DATA_BLOCK "IMAC_TANK_RECORD"
TITLE = TANK_RECORD
AUTHOR : HottendU
FAMILY : IMAC
VERSION : 0.2


  STRUCT
   TANK_No001 : STRUCT
    PCONF : STRUCT
     ObjInput : INT  := 1511;	//IMAC L (AvEdit) Objectnumber of pressure/level transmitter, Unit [m] or [bar]
     ObjTemp : INT  := 1512;	//IMAC L (AvEdit) Objectnumber of temperature transmitter
     SklRefNo : BYTE  := B#16#2;	//IMAC L Scaling Group No (AvEdit) user for Tank Table (x=Level, y=Volume)
     Offset : REAL ;	//Offset of pressure transmitter from bottom of tank
     LL_XTsub : REAL ;	//Low limit operator input tank temperature
     HL_XTsub : REAL  := 1.500000e+002;	//High limit operator input tank temperature
     LL_XDensity : REAL ;	//Low limit operator input density (t ref)
     HL_XDensity : REAL  := 5.000000e+000;	//High limit operator input density (t ref)
     LL_XRefTemp : REAL ;	//Low limit operator input reference temperature
     HL_XRefTemp : REAL  := 1.500000e+002;	//High limit operator input reference temperature
     LL_XVEC : REAL ;	//Low limit operator input volume expansion coefficiency
     HL_XVEC : REAL  := 5.000000e+000;	//High limit operator input volume expansion coefficiency
     Modeswitches : STRUCT
      M0_SensorConfiguration : BOOL ;	// 0: Pressure Sensor;  1: Level Sensor
      M1_TemperatureComp : BOOL  := TRUE;	// 0: without Compensation;   1: with compensation
      M2 : BOOL ;	//
      M3 : BOOL ;	//
      M4 : BOOL ;	//
      M5 : BOOL ;	//
      M6 : BOOL ;
      M7 : BOOL ;	//
      M8 : BOOL ;	//
      M9 : BOOL ;	//
      M10 : BOOL ;
      M11 : BOOL ;
      M12 : BOOL ;
      M13 : BOOL ;
      M14 : BOOL ;
      M15 : BOOL ;	//
     END_STRUCT ;
    END_STRUCT ;
   END_STRUCT ;
   TANK_No002 : STRUCT
    PCONF : STRUCT
     ObjInput : INT ;	//IMAC L (AvEdit) Objectnumber of pressure/level transmitter, Unit [m] or [bar]
     ObjTemp : INT ;	//IMAC L (AvEdit) Objectnumber of temperature transmitter
     SklRefNo : BYTE ;	//IMAC L Scaling Group No (AvEdit) user for Tank Table (x=Level, y=Volume)
     Offset : REAL ;	//Offset of pressure transmitter from bottom of tank
     LL_XTsub : REAL ;	//Low limit operator input tank temperature
     HL_XTsub : REAL  := 1.500000e+002;	//High limit operator input tank temperature
     LL_XDensity : REAL ;	//Low limit operator input density (t ref)
     HL_XDensity : REAL  := 5.000000e+000;	//High limit operator input density (t ref)
     LL_XRefTemp : REAL ;	//Low limit operator input reference temperature
     HL_XRefTemp : REAL  := 1.500000e+002;	//High limit operator input reference temperature
     LL_XVEC : REAL ;	//Low limit operator input volume expansion coefficiency
     HL_XVEC : REAL  := 5.000000e+000;	//High limit operator input volume expansion coefficiency
     Modeswitches : STRUCT
      M0_SensorConfiguration : BOOL ;	// 0: Pressure Sensor;  1: Level Sensor
      M1_TemperatureComp : BOOL ;	// 0: without Compensation;   1: with compensation
      M2 : BOOL ;	//
      M3 : BOOL ;	//
      M4 : BOOL ;	//
      M5 : BOOL ;	//
      M6 : BOOL ;
      M7 : BOOL ;	//
      M8 : BOOL ;	//
      M9 : BOOL ;	//
      M10 : BOOL ;
      M11 : BOOL ;
      M12 : BOOL ;
      M13 : BOOL ;
      M14 : BOOL ;
      M15 : BOOL ;	//
     END_STRUCT ;
    END_STRUCT ;
   END_STRUCT ;
   TANK_No003 : STRUCT
    PCONF : STRUCT
     ObjInput : INT ;	//IMAC L (AvEdit) Objectnumber of pressure/level transmitter, Unit [m] or [bar]
     ObjTemp : INT ;	//IMAC L (AvEdit) Objectnumber of temperature transmitter
     SklRefNo : BYTE ;	//IMAC L Scaling Group No (AvEdit) user for Tank Table (x=Level, y=Volume)
     Offset : REAL ;	//Offset of pressure transmitter from bottom of tank
     LL_XTsub : REAL ;	//Low limit operator input tank temperature
     HL_XTsub : REAL  := 1.500000e+002;	//High limit operator input tank temperature
     LL_XDensity : REAL ;	//Low limit operator input density (t ref)
     HL_XDensity : REAL  := 5.000000e+000;	//High limit operator input density (t ref)
     LL_XRefTemp : REAL ;	//Low limit operator input reference temperature
     HL_XRefTemp : REAL  := 1.500000e+002;	//High limit operator input reference temperature
     LL_XVEC : REAL ;	//Low limit operator input volume expansion coefficiency
     HL_XVEC : REAL  := 5.000000e+000;	//High limit operator input volume expansion coefficiency
     Modeswitches : STRUCT
      M0_SensorConfiguration : BOOL ;	// 0: Pressure Sensor;  1: Level Sensor
      M1_TemperatureComp : BOOL ;	// 0: without Compensation;   1: with compensation
      M2 : BOOL ;	//
      M3 : BOOL ;	//
      M4 : BOOL ;	//
      M5 : BOOL ;	//
      M6 : BOOL ;
      M7 : BOOL ;	//
      M8 : BOOL ;	//
      M9 : BOOL ;	//
      M10 : BOOL ;
      M11 : BOOL ;
      M12 : BOOL ;
      M13 : BOOL ;
      M14 : BOOL ;
      M15 : BOOL ;	//
     END_STRUCT ;
    END_STRUCT ;
   END_STRUCT ;
   TANK_No004 : STRUCT
    PCONF : STRUCT
     ObjInput : INT ;	//IMAC L (AvEdit) Objectnumber of pressure/level transmitter, Unit [m] or [bar]
     ObjTemp : INT ;	//IMAC L (AvEdit) Objectnumber of temperature transmitter
     SklRefNo : BYTE ;	//IMAC L Scaling Group No (AvEdit) user for Tank Table (x=Level, y=Volume)
     Offset : REAL ;	//Offset of pressure transmitter from bottom of tank
     LL_XTsub : REAL ;	//Low limit operator input tank temperature
     HL_XTsub : REAL  := 1.500000e+002;	//High limit operator input tank temperature
     LL_XDensity : REAL ;	//Low limit operator input density (t ref)
     HL_XDensity : REAL  := 5.000000e+000;	//High limit operator input density (t ref)
     LL_XRefTemp : REAL ;	//Low limit operator input reference temperature
     HL_XRefTemp : REAL  := 1.500000e+002;	//High limit operator input reference temperature
     LL_XVEC : REAL ;	//Low limit operator input volume expansion coefficiency
     HL_XVEC : REAL  := 5.000000e+000;	//High limit operator input volume expansion coefficiency
     Modeswitches : STRUCT
      M0_SensorConfiguration : BOOL ;	// 0: Pressure Sensor;  1: Level Sensor
      M1_TemperatureComp : BOOL ;	// 0: without Compensation;   1: with compensation
      M2 : BOOL ;	//
      M3 : BOOL ;	//
      M4 : BOOL ;	//
      M5 : BOOL ;	//
      M6 : BOOL ;
      M7 : BOOL ;	//
      M8 : BOOL ;	//
      M9 : BOOL ;	//
      M10 : BOOL ;
      M11 : BOOL ;
      M12 : BOOL ;
      M13 : BOOL ;
      M14 : BOOL ;
      M15 : BOOL ;	//
     END_STRUCT ;
    END_STRUCT ;
   END_STRUCT ;
   TANK_No005 : STRUCT
    PCONF : STRUCT
     ObjInput : INT ;	//IMAC L (AvEdit) Objectnumber of pressure/level transmitter, Unit [m] or [bar]
     ObjTemp : INT ;	//IMAC L (AvEdit) Objectnumber of temperature transmitter
     SklRefNo : BYTE ;	//IMAC L Scaling Group No (AvEdit) user for Tank Table (x=Level, y=Volume)
     Offset : REAL ;	//Offset of pressure transmitter from bottom of tank
     LL_XTsub : REAL ;	//Low limit operator input tank temperature
     HL_XTsub : REAL  := 1.500000e+002;	//High limit operator input tank temperature
     LL_XDensity : REAL ;	//Low limit operator input density (t ref)
     HL_XDensity : REAL  := 5.000000e+000;	//High limit operator input density (t ref)
     LL_XRefTemp : REAL ;	//Low limit operator input reference temperature
     HL_XRefTemp : REAL  := 1.500000e+002;	//High limit operator input reference temperature
     LL_XVEC : REAL ;	//Low limit operator input volume expansion coefficiency
     HL_XVEC : REAL  := 5.000000e+000;	//High limit operator input volume expansion coefficiency
     Modeswitches : STRUCT
      M0_SensorConfiguration : BOOL ;	// 0: Pressure Sensor;  1: Level Sensor
      M1_TemperatureComp : BOOL ;	// 0: without Compensation;   1: with compensation
      M2 : BOOL ;	//
      M3 : BOOL ;	//
      M4 : BOOL ;	//
      M5 : BOOL ;	//
      M6 : BOOL ;
      M7 : BOOL ;	//
      M8 : BOOL ;	//
      M9 : BOOL ;	//
      M10 : BOOL ;
      M11 : BOOL ;
      M12 : BOOL ;
      M13 : BOOL ;
      M14 : BOOL ;
      M15 : BOOL ;	//
     END_STRUCT ;
    END_STRUCT ;
   END_STRUCT ;
   TANK_No006 : STRUCT
    PCONF : STRUCT
     ObjInput : INT ;	//IMAC L (AvEdit) Objectnumber of pressure/level transmitter, Unit [m] or [bar]
     ObjTemp : INT ;	//IMAC L (AvEdit) Objectnumber of temperature transmitter
     SklRefNo : BYTE ;	//IMAC L Scaling Group No (AvEdit) user for Tank Table (x=Level, y=Volume)
     Offset : REAL ;	//Offset of pressure transmitter from bottom of tank
     LL_XTsub : REAL ;	//Low limit operator input tank temperature
     HL_XTsub : REAL  := 1.500000e+002;	//High limit operator input tank temperature
     LL_XDensity : REAL ;	//Low limit operator input density (t ref)
     HL_XDensity : REAL  := 5.000000e+000;	//High limit operator input density (t ref)
     LL_XRefTemp : REAL ;	//Low limit operator input reference temperature
     HL_XRefTemp : REAL  := 1.500000e+002;	//High limit operator input reference temperature
     LL_XVEC : REAL ;	//Low limit operator input volume expansion coefficiency
     HL_XVEC : REAL  := 5.000000e+000;	//High limit operator input volume expansion coefficiency
     Modeswitches : STRUCT
      M0_SensorConfiguration : BOOL ;	// 0: Pressure Sensor;  1: Level Sensor
      M1_TemperatureComp : BOOL ;	// 0: without Compensation;   1: with compensation
      M2 : BOOL ;	//
      M3 : BOOL ;	//
      M4 : BOOL ;	//
      M5 : BOOL ;	//
      M6 : BOOL ;
      M7 : BOOL ;	//
      M8 : BOOL ;	//
      M9 : BOOL ;	//
      M10 : BOOL ;
      M11 : BOOL ;
      M12 : BOOL ;
      M13 : BOOL ;
      M14 : BOOL ;
      M15 : BOOL ;	//
     END_STRUCT ;
    END_STRUCT ;
   END_STRUCT ;
   TANK_No007 : STRUCT
    PCONF : STRUCT
     ObjInput : INT ;	//IMAC L (AvEdit) Objectnumber of pressure/level transmitter, Unit [m] or [bar]
     ObjTemp : INT ;	//IMAC L (AvEdit) Objectnumber of temperature transmitter
     SklRefNo : BYTE ;	//IMAC L Scaling Group No (AvEdit) user for Tank Table (x=Level, y=Volume)
     Offset : REAL ;	//Offset of pressure transmitter from bottom of tank
     LL_XTsub : REAL ;	//Low limit operator input tank temperature
     HL_XTsub : REAL  := 1.500000e+002;	//High limit operator input tank temperature
     LL_XDensity : REAL ;	//Low limit operator input density (t ref)
     HL_XDensity : REAL  := 5.000000e+000;	//High limit operator input density (t ref)
     LL_XRefTemp : REAL ;	//Low limit operator input reference temperature
     HL_XRefTemp : REAL  := 1.500000e+002;	//High limit operator input reference temperature
     LL_XVEC : REAL ;	//Low limit operator input volume expansion coefficiency
     HL_XVEC : REAL  := 5.000000e+000;	//High limit operator input volume expansion coefficiency
     Modeswitches : STRUCT
      M0_SensorConfiguration : BOOL ;	// 0: Pressure Sensor;  1: Level Sensor
      M1_TemperatureComp : BOOL ;	// 0: without Compensation;   1: with compensation
      M2 : BOOL ;	//
      M3 : BOOL ;	//
      M4 : BOOL ;	//
      M5 : BOOL ;	//
      M6 : BOOL ;
      M7 : BOOL ;	//
      M8 : BOOL ;	//
      M9 : BOOL ;	//
      M10 : BOOL ;
      M11 : BOOL ;
      M12 : BOOL ;
      M13 : BOOL ;
      M14 : BOOL ;
      M15 : BOOL ;	//
     END_STRUCT ;
    END_STRUCT ;
   END_STRUCT ;
   TANK_No008 : STRUCT
    PCONF : STRUCT
     ObjInput : INT ;	//IMAC L (AvEdit) Objectnumber of pressure/level transmitter, Unit [m] or [bar]
     ObjTemp : INT ;	//IMAC L (AvEdit) Objectnumber of temperature transmitter
     SklRefNo : BYTE ;	//IMAC L Scaling Group No (AvEdit) user for Tank Table (x=Level, y=Volume)
     Offset : REAL ;	//Offset of pressure transmitter from bottom of tank
     LL_XTsub : REAL ;	//Low limit operator input tank temperature
     HL_XTsub : REAL  := 1.500000e+002;	//High limit operator input tank temperature
     LL_XDensity : REAL ;	//Low limit operator input density (t ref)
     HL_XDensity : REAL  := 5.000000e+000;	//High limit operator input density (t ref)
     LL_XRefTemp : REAL ;	//Low limit operator input reference temperature
     HL_XRefTemp : REAL  := 1.500000e+002;	//High limit operator input reference temperature
     LL_XVEC : REAL ;	//Low limit operator input volume expansion coefficiency
     HL_XVEC : REAL  := 5.000000e+000;	//High limit operator input volume expansion coefficiency
     Modeswitches : STRUCT
      M0_SensorConfiguration : BOOL ;	// 0: Pressure Sensor;  1: Level Sensor
      M1_TemperatureComp : BOOL ;	// 0: without Compensation;   1: with compensation
      M2 : BOOL ;	//
      M3 : BOOL ;	//
      M4 : BOOL ;	//
      M5 : BOOL ;	//
      M6 : BOOL ;
      M7 : BOOL ;	//
      M8 : BOOL ;	//
      M9 : BOOL ;	//
      M10 : BOOL ;
      M11 : BOOL ;
      M12 : BOOL ;
      M13 : BOOL ;
      M14 : BOOL ;
      M15 : BOOL ;	//
     END_STRUCT ;
    END_STRUCT ;
   END_STRUCT ;
   TANK_No009 : STRUCT
    PCONF : STRUCT
     ObjInput : INT ;	//IMAC L (AvEdit) Objectnumber of pressure/level transmitter, Unit [m] or [bar]
     ObjTemp : INT ;	//IMAC L (AvEdit) Objectnumber of temperature transmitter
     SklRefNo : BYTE ;	//IMAC L Scaling Group No (AvEdit) user for Tank Table (x=Level, y=Volume)
     Offset : REAL ;	//Offset of pressure transmitter from bottom of tank
     LL_XTsub : REAL ;	//Low limit operator input tank temperature
     HL_XTsub : REAL  := 1.500000e+002;	//High limit operator input tank temperature
     LL_XDensity : REAL ;	//Low limit operator input density (t ref)
     HL_XDensity : REAL  := 5.000000e+000;	//High limit operator input density (t ref)
     LL_XRefTemp : REAL ;	//Low limit operator input reference temperature
     HL_XRefTemp : REAL  := 1.500000e+002;	//High limit operator input reference temperature
     LL_XVEC : REAL ;	//Low limit operator input volume expansion coefficiency
     HL_XVEC : REAL  := 5.000000e+000;	//High limit operator input volume expansion coefficiency
     Modeswitches : STRUCT
      M0_SensorConfiguration : BOOL ;	// 0: Pressure Sensor;  1: Level Sensor
      M1_TemperatureComp : BOOL ;	// 0: without Compensation;   1: with compensation
      M2 : BOOL ;	//
      M3 : BOOL ;	//
      M4 : BOOL ;	//
      M5 : BOOL ;	//
      M6 : BOOL ;
      M7 : BOOL ;	//
      M8 : BOOL ;	//
      M9 : BOOL ;	//
      M10 : BOOL ;
      M11 : BOOL ;
      M12 : BOOL ;
      M13 : BOOL ;
      M14 : BOOL ;
      M15 : BOOL ;	//
     END_STRUCT ;
    END_STRUCT ;
   END_STRUCT ;
   TANK_No0010 : STRUCT
    PCONF : STRUCT
     ObjInput : INT ;	//IMAC L (AvEdit) Objectnumber of pressure/level transmitter, Unit [m] or [bar]
     ObjTemp : INT ;	//IMAC L (AvEdit) Objectnumber of temperature transmitter
     SklRefNo : BYTE ;	//IMAC L Scaling Group No (AvEdit) user for Tank Table (x=Level, y=Volume)
     Offset : REAL ;	//Offset of pressure transmitter from bottom of tank
     LL_XTsub : REAL ;	//Low limit operator input tank temperature
     HL_XTsub : REAL  := 1.500000e+002;	//High limit operator input tank temperature
     LL_XDensity : REAL ;	//Low limit operator input density (t ref)
     HL_XDensity : REAL  := 5.000000e+000;	//High limit operator input density (t ref)
     LL_XRefTemp : REAL ;	//Low limit operator input reference temperature
     HL_XRefTemp : REAL  := 1.500000e+002;	//High limit operator input reference temperature
     LL_XVEC : REAL ;	//Low limit operator input volume expansion coefficiency
     HL_XVEC : REAL  := 5.000000e+000;	//High limit operator input volume expansion coefficiency
     Modeswitches : STRUCT
      M0_SensorConfiguration : BOOL ;	// 0: Pressure Sensor;  1: Level Sensor
      M1_TemperatureComp : BOOL ;	// 0: without Compensation;   1: with compensation
      M2 : BOOL ;	//
      M3 : BOOL ;	//
      M4 : BOOL ;	//
      M5 : BOOL ;	//
      M6 : BOOL ;
      M7 : BOOL ;	//
      M8 : BOOL ;	//
      M9 : BOOL ;	//
      M10 : BOOL ;
      M11 : BOOL ;
      M12 : BOOL ;
      M13 : BOOL ;
      M14 : BOOL ;
      M15 : BOOL ;	//
     END_STRUCT ;
    END_STRUCT ;
   END_STRUCT ;
  END_STRUCT ;
BEGIN
   TANK_No001.PCONF.ObjInput := 1511;
   TANK_No001.PCONF.ObjTemp := 1512;
   TANK_No001.PCONF.SklRefNo := B#16#2;
   TANK_No001.PCONF.Offset := 0.000000e+000;
   TANK_No001.PCONF.LL_XTsub := 0.000000e+000;
   TANK_No001.PCONF.HL_XTsub := 1.500000e+002;
   TANK_No001.PCONF.LL_XDensity := 0.000000e+000;
   TANK_No001.PCONF.HL_XDensity := 5.000000e+000;
   TANK_No001.PCONF.LL_XRefTemp := 0.000000e+000;
   TANK_No001.PCONF.HL_XRefTemp := 1.500000e+002;
   TANK_No001.PCONF.LL_XVEC := 0.000000e+000;
   TANK_No001.PCONF.HL_XVEC := 5.000000e+000;
   TANK_No001.PCONF.Modeswitches.M0_SensorConfiguration := FALSE;
   TANK_No001.PCONF.Modeswitches.M1_TemperatureComp := TRUE;
   TANK_No001.PCONF.Modeswitches.M2 := FALSE;
   TANK_No001.PCONF.Modeswitches.M3 := FALSE;
   TANK_No001.PCONF.Modeswitches.M4 := FALSE;
   TANK_No001.PCONF.Modeswitches.M5 := FALSE;
   TANK_No001.PCONF.Modeswitches.M6 := FALSE;
   TANK_No001.PCONF.Modeswitches.M7 := FALSE;
   TANK_No001.PCONF.Modeswitches.M8 := FALSE;
   TANK_No001.PCONF.Modeswitches.M9 := FALSE;
   TANK_No001.PCONF.Modeswitches.M10 := FALSE;
   TANK_No001.PCONF.Modeswitches.M11 := FALSE;
   TANK_No001.PCONF.Modeswitches.M12 := FALSE;
   TANK_No001.PCONF.Modeswitches.M13 := FALSE;
   TANK_No001.PCONF.Modeswitches.M14 := FALSE;
   TANK_No001.PCONF.Modeswitches.M15 := FALSE;
   TANK_No002.PCONF.ObjInput := 0;
   TANK_No002.PCONF.ObjTemp := 0;
   TANK_No002.PCONF.SklRefNo := B#16#0;
   TANK_No002.PCONF.Offset := 0.000000e+000;
   TANK_No002.PCONF.LL_XTsub := 0.000000e+000;
   TANK_No002.PCONF.HL_XTsub := 1.500000e+002;
   TANK_No002.PCONF.LL_XDensity := 0.000000e+000;
   TANK_No002.PCONF.HL_XDensity := 5.000000e+000;
   TANK_No002.PCONF.LL_XRefTemp := 0.000000e+000;
   TANK_No002.PCONF.HL_XRefTemp := 1.500000e+002;
   TANK_No002.PCONF.LL_XVEC := 0.000000e+000;
   TANK_No002.PCONF.HL_XVEC := 5.000000e+000;
   TANK_No002.PCONF.Modeswitches.M0_SensorConfiguration := FALSE;
   TANK_No002.PCONF.Modeswitches.M1_TemperatureComp := FALSE;
   TANK_No002.PCONF.Modeswitches.M2 := FALSE;
   TANK_No002.PCONF.Modeswitches.M3 := FALSE;
   TANK_No002.PCONF.Modeswitches.M4 := FALSE;
   TANK_No002.PCONF.Modeswitches.M5 := FALSE;
   TANK_No002.PCONF.Modeswitches.M6 := FALSE;
   TANK_No002.PCONF.Modeswitches.M7 := FALSE;
   TANK_No002.PCONF.Modeswitches.M8 := FALSE;
   TANK_No002.PCONF.Modeswitches.M9 := FALSE;
   TANK_No002.PCONF.Modeswitches.M10 := FALSE;
   TANK_No002.PCONF.Modeswitches.M11 := FALSE;
   TANK_No002.PCONF.Modeswitches.M12 := FALSE;
   TANK_No002.PCONF.Modeswitches.M13 := FALSE;
   TANK_No002.PCONF.Modeswitches.M14 := FALSE;
   TANK_No002.PCONF.Modeswitches.M15 := FALSE;
   TANK_No003.PCONF.ObjInput := 0;
   TANK_No003.PCONF.ObjTemp := 0;
   TANK_No003.PCONF.SklRefNo := B#16#0;
   TANK_No003.PCONF.Offset := 0.000000e+000;
   TANK_No003.PCONF.LL_XTsub := 0.000000e+000;
   TANK_No003.PCONF.HL_XTsub := 1.500000e+002;
   TANK_No003.PCONF.LL_XDensity := 0.000000e+000;
   TANK_No003.PCONF.HL_XDensity := 5.000000e+000;
   TANK_No003.PCONF.LL_XRefTemp := 0.000000e+000;
   TANK_No003.PCONF.HL_XRefTemp := 1.500000e+002;
   TANK_No003.PCONF.LL_XVEC := 0.000000e+000;
   TANK_No003.PCONF.HL_XVEC := 5.000000e+000;
   TANK_No003.PCONF.Modeswitches.M0_SensorConfiguration := FALSE;
   TANK_No003.PCONF.Modeswitches.M1_TemperatureComp := FALSE;
   TANK_No003.PCONF.Modeswitches.M2 := FALSE;
   TANK_No003.PCONF.Modeswitches.M3 := FALSE;
   TANK_No003.PCONF.Modeswitches.M4 := FALSE;
   TANK_No003.PCONF.Modeswitches.M5 := FALSE;
   TANK_No003.PCONF.Modeswitches.M6 := FALSE;
   TANK_No003.PCONF.Modeswitches.M7 := FALSE;
   TANK_No003.PCONF.Modeswitches.M8 := FALSE;
   TANK_No003.PCONF.Modeswitches.M9 := FALSE;
   TANK_No003.PCONF.Modeswitches.M10 := FALSE;
   TANK_No003.PCONF.Modeswitches.M11 := FALSE;
   TANK_No003.PCONF.Modeswitches.M12 := FALSE;
   TANK_No003.PCONF.Modeswitches.M13 := FALSE;
   TANK_No003.PCONF.Modeswitches.M14 := FALSE;
   TANK_No003.PCONF.Modeswitches.M15 := FALSE;
   TANK_No004.PCONF.ObjInput := 0;
   TANK_No004.PCONF.ObjTemp := 0;
   TANK_No004.PCONF.SklRefNo := B#16#0;
   TANK_No004.PCONF.Offset := 0.000000e+000;
   TANK_No004.PCONF.LL_XTsub := 0.000000e+000;
   TANK_No004.PCONF.HL_XTsub := 1.500000e+002;
   TANK_No004.PCONF.LL_XDensity := 0.000000e+000;
   TANK_No004.PCONF.HL_XDensity := 5.000000e+000;
   TANK_No004.PCONF.LL_XRefTemp := 0.000000e+000;
   TANK_No004.PCONF.HL_XRefTemp := 1.500000e+002;
   TANK_No004.PCONF.LL_XVEC := 0.000000e+000;
   TANK_No004.PCONF.HL_XVEC := 5.000000e+000;
   TANK_No004.PCONF.Modeswitches.M0_SensorConfiguration := FALSE;
   TANK_No004.PCONF.Modeswitches.M1_TemperatureComp := FALSE;
   TANK_No004.PCONF.Modeswitches.M2 := FALSE;
   TANK_No004.PCONF.Modeswitches.M3 := FALSE;
   TANK_No004.PCONF.Modeswitches.M4 := FALSE;
   TANK_No004.PCONF.Modeswitches.M5 := FALSE;
   TANK_No004.PCONF.Modeswitches.M6 := FALSE;
   TANK_No004.PCONF.Modeswitches.M7 := FALSE;
   TANK_No004.PCONF.Modeswitches.M8 := FALSE;
   TANK_No004.PCONF.Modeswitches.M9 := FALSE;
   TANK_No004.PCONF.Modeswitches.M10 := FALSE;
   TANK_No004.PCONF.Modeswitches.M11 := FALSE;
   TANK_No004.PCONF.Modeswitches.M12 := FALSE;
   TANK_No004.PCONF.Modeswitches.M13 := FALSE;
   TANK_No004.PCONF.Modeswitches.M14 := FALSE;
   TANK_No004.PCONF.Modeswitches.M15 := FALSE;
   TANK_No005.PCONF.ObjInput := 0;
   TANK_No005.PCONF.ObjTemp := 0;
   TANK_No005.PCONF.SklRefNo := B#16#0;
   TANK_No005.PCONF.Offset := 0.000000e+000;
   TANK_No005.PCONF.LL_XTsub := 0.000000e+000;
   TANK_No005.PCONF.HL_XTsub := 1.500000e+002;
   TANK_No005.PCONF.LL_XDensity := 0.000000e+000;
   TANK_No005.PCONF.HL_XDensity := 5.000000e+000;
   TANK_No005.PCONF.LL_XRefTemp := 0.000000e+000;
   TANK_No005.PCONF.HL_XRefTemp := 1.500000e+002;
   TANK_No005.PCONF.LL_XVEC := 0.000000e+000;
   TANK_No005.PCONF.HL_XVEC := 5.000000e+000;
   TANK_No005.PCONF.Modeswitches.M0_SensorConfiguration := FALSE;
   TANK_No005.PCONF.Modeswitches.M1_TemperatureComp := FALSE;
   TANK_No005.PCONF.Modeswitches.M2 := FALSE;
   TANK_No005.PCONF.Modeswitches.M3 := FALSE;
   TANK_No005.PCONF.Modeswitches.M4 := FALSE;
   TANK_No005.PCONF.Modeswitches.M5 := FALSE;
   TANK_No005.PCONF.Modeswitches.M6 := FALSE;
   TANK_No005.PCONF.Modeswitches.M7 := FALSE;
   TANK_No005.PCONF.Modeswitches.M8 := FALSE;
   TANK_No005.PCONF.Modeswitches.M9 := FALSE;
   TANK_No005.PCONF.Modeswitches.M10 := FALSE;
   TANK_No005.PCONF.Modeswitches.M11 := FALSE;
   TANK_No005.PCONF.Modeswitches.M12 := FALSE;
   TANK_No005.PCONF.Modeswitches.M13 := FALSE;
   TANK_No005.PCONF.Modeswitches.M14 := FALSE;
   TANK_No005.PCONF.Modeswitches.M15 := FALSE;
   TANK_No006.PCONF.ObjInput := 0;
   TANK_No006.PCONF.ObjTemp := 0;
   TANK_No006.PCONF.SklRefNo := B#16#0;
   TANK_No006.PCONF.Offset := 0.000000e+000;
   TANK_No006.PCONF.LL_XTsub := 0.000000e+000;
   TANK_No006.PCONF.HL_XTsub := 1.500000e+002;
   TANK_No006.PCONF.LL_XDensity := 0.000000e+000;
   TANK_No006.PCONF.HL_XDensity := 5.000000e+000;
   TANK_No006.PCONF.LL_XRefTemp := 0.000000e+000;
   TANK_No006.PCONF.HL_XRefTemp := 1.500000e+002;
   TANK_No006.PCONF.LL_XVEC := 0.000000e+000;
   TANK_No006.PCONF.HL_XVEC := 5.000000e+000;
   TANK_No006.PCONF.Modeswitches.M0_SensorConfiguration := FALSE;
   TANK_No006.PCONF.Modeswitches.M1_TemperatureComp := FALSE;
   TANK_No006.PCONF.Modeswitches.M2 := FALSE;
   TANK_No006.PCONF.Modeswitches.M3 := FALSE;
   TANK_No006.PCONF.Modeswitches.M4 := FALSE;
   TANK_No006.PCONF.Modeswitches.M5 := FALSE;
   TANK_No006.PCONF.Modeswitches.M6 := FALSE;
   TANK_No006.PCONF.Modeswitches.M7 := FALSE;
   TANK_No006.PCONF.Modeswitches.M8 := FALSE;
   TANK_No006.PCONF.Modeswitches.M9 := FALSE;
   TANK_No006.PCONF.Modeswitches.M10 := FALSE;
   TANK_No006.PCONF.Modeswitches.M11 := FALSE;
   TANK_No006.PCONF.Modeswitches.M12 := FALSE;
   TANK_No006.PCONF.Modeswitches.M13 := FALSE;
   TANK_No006.PCONF.Modeswitches.M14 := FALSE;
   TANK_No006.PCONF.Modeswitches.M15 := FALSE;
   TANK_No007.PCONF.ObjInput := 0;
   TANK_No007.PCONF.ObjTemp := 0;
   TANK_No007.PCONF.SklRefNo := B#16#0;
   TANK_No007.PCONF.Offset := 0.000000e+000;
   TANK_No007.PCONF.LL_XTsub := 0.000000e+000;
   TANK_No007.PCONF.HL_XTsub := 1.500000e+002;
   TANK_No007.PCONF.LL_XDensity := 0.000000e+000;
   TANK_No007.PCONF.HL_XDensity := 5.000000e+000;
   TANK_No007.PCONF.LL_XRefTemp := 0.000000e+000;
   TANK_No007.PCONF.HL_XRefTemp := 1.500000e+002;
   TANK_No007.PCONF.LL_XVEC := 0.000000e+000;
   TANK_No007.PCONF.HL_XVEC := 5.000000e+000;
   TANK_No007.PCONF.Modeswitches.M0_SensorConfiguration := FALSE;
   TANK_No007.PCONF.Modeswitches.M1_TemperatureComp := FALSE;
   TANK_No007.PCONF.Modeswitches.M2 := FALSE;
   TANK_No007.PCONF.Modeswitches.M3 := FALSE;
   TANK_No007.PCONF.Modeswitches.M4 := FALSE;
   TANK_No007.PCONF.Modeswitches.M5 := FALSE;
   TANK_No007.PCONF.Modeswitches.M6 := FALSE;
   TANK_No007.PCONF.Modeswitches.M7 := FALSE;
   TANK_No007.PCONF.Modeswitches.M8 := FALSE;
   TANK_No007.PCONF.Modeswitches.M9 := FALSE;
   TANK_No007.PCONF.Modeswitches.M10 := FALSE;
   TANK_No007.PCONF.Modeswitches.M11 := FALSE;
   TANK_No007.PCONF.Modeswitches.M12 := FALSE;
   TANK_No007.PCONF.Modeswitches.M13 := FALSE;
   TANK_No007.PCONF.Modeswitches.M14 := FALSE;
   TANK_No007.PCONF.Modeswitches.M15 := FALSE;
   TANK_No008.PCONF.ObjInput := 0;
   TANK_No008.PCONF.ObjTemp := 0;
   TANK_No008.PCONF.SklRefNo := B#16#0;
   TANK_No008.PCONF.Offset := 0.000000e+000;
   TANK_No008.PCONF.LL_XTsub := 0.000000e+000;
   TANK_No008.PCONF.HL_XTsub := 1.500000e+002;
   TANK_No008.PCONF.LL_XDensity := 0.000000e+000;
   TANK_No008.PCONF.HL_XDensity := 5.000000e+000;
   TANK_No008.PCONF.LL_XRefTemp := 0.000000e+000;
   TANK_No008.PCONF.HL_XRefTemp := 1.500000e+002;
   TANK_No008.PCONF.LL_XVEC := 0.000000e+000;
   TANK_No008.PCONF.HL_XVEC := 5.000000e+000;
   TANK_No008.PCONF.Modeswitches.M0_SensorConfiguration := FALSE;
   TANK_No008.PCONF.Modeswitches.M1_TemperatureComp := FALSE;
   TANK_No008.PCONF.Modeswitches.M2 := FALSE;
   TANK_No008.PCONF.Modeswitches.M3 := FALSE;
   TANK_No008.PCONF.Modeswitches.M4 := FALSE;
   TANK_No008.PCONF.Modeswitches.M5 := FALSE;
   TANK_No008.PCONF.Modeswitches.M6 := FALSE;
   TANK_No008.PCONF.Modeswitches.M7 := FALSE;
   TANK_No008.PCONF.Modeswitches.M8 := FALSE;
   TANK_No008.PCONF.Modeswitches.M9 := FALSE;
   TANK_No008.PCONF.Modeswitches.M10 := FALSE;
   TANK_No008.PCONF.Modeswitches.M11 := FALSE;
   TANK_No008.PCONF.Modeswitches.M12 := FALSE;
   TANK_No008.PCONF.Modeswitches.M13 := FALSE;
   TANK_No008.PCONF.Modeswitches.M14 := FALSE;
   TANK_No008.PCONF.Modeswitches.M15 := FALSE;
   TANK_No009.PCONF.ObjInput := 0;
   TANK_No009.PCONF.ObjTemp := 0;
   TANK_No009.PCONF.SklRefNo := B#16#0;
   TANK_No009.PCONF.Offset := 0.000000e+000;
   TANK_No009.PCONF.LL_XTsub := 0.000000e+000;
   TANK_No009.PCONF.HL_XTsub := 1.500000e+002;
   TANK_No009.PCONF.LL_XDensity := 0.000000e+000;
   TANK_No009.PCONF.HL_XDensity := 5.000000e+000;
   TANK_No009.PCONF.LL_XRefTemp := 0.000000e+000;
   TANK_No009.PCONF.HL_XRefTemp := 1.500000e+002;
   TANK_No009.PCONF.LL_XVEC := 0.000000e+000;
   TANK_No009.PCONF.HL_XVEC := 5.000000e+000;
   TANK_No009.PCONF.Modeswitches.M0_SensorConfiguration := FALSE;
   TANK_No009.PCONF.Modeswitches.M1_TemperatureComp := FALSE;
   TANK_No009.PCONF.Modeswitches.M2 := FALSE;
   TANK_No009.PCONF.Modeswitches.M3 := FALSE;
   TANK_No009.PCONF.Modeswitches.M4 := FALSE;
   TANK_No009.PCONF.Modeswitches.M5 := FALSE;
   TANK_No009.PCONF.Modeswitches.M6 := FALSE;
   TANK_No009.PCONF.Modeswitches.M7 := FALSE;
   TANK_No009.PCONF.Modeswitches.M8 := FALSE;
   TANK_No009.PCONF.Modeswitches.M9 := FALSE;
   TANK_No009.PCONF.Modeswitches.M10 := FALSE;
   TANK_No009.PCONF.Modeswitches.M11 := FALSE;
   TANK_No009.PCONF.Modeswitches.M12 := FALSE;
   TANK_No009.PCONF.Modeswitches.M13 := FALSE;
   TANK_No009.PCONF.Modeswitches.M14 := FALSE;
   TANK_No009.PCONF.Modeswitches.M15 := FALSE;
   TANK_No0010.PCONF.ObjInput := 0;
   TANK_No0010.PCONF.ObjTemp := 0;
   TANK_No0010.PCONF.SklRefNo := B#16#0;
   TANK_No0010.PCONF.Offset := 0.000000e+000;
   TANK_No0010.PCONF.LL_XTsub := 0.000000e+000;
   TANK_No0010.PCONF.HL_XTsub := 1.500000e+002;
   TANK_No0010.PCONF.LL_XDensity := 0.000000e+000;
   TANK_No0010.PCONF.HL_XDensity := 5.000000e+000;
   TANK_No0010.PCONF.LL_XRefTemp := 0.000000e+000;
   TANK_No0010.PCONF.HL_XRefTemp := 1.500000e+002;
   TANK_No0010.PCONF.LL_XVEC := 0.000000e+000;
   TANK_No0010.PCONF.HL_XVEC := 5.000000e+000;
   TANK_No0010.PCONF.Modeswitches.M0_SensorConfiguration := FALSE;
   TANK_No0010.PCONF.Modeswitches.M1_TemperatureComp := FALSE;
   TANK_No0010.PCONF.Modeswitches.M2 := FALSE;
   TANK_No0010.PCONF.Modeswitches.M3 := FALSE;
   TANK_No0010.PCONF.Modeswitches.M4 := FALSE;
   TANK_No0010.PCONF.Modeswitches.M5 := FALSE;
   TANK_No0010.PCONF.Modeswitches.M6 := FALSE;
   TANK_No0010.PCONF.Modeswitches.M7 := FALSE;
   TANK_No0010.PCONF.Modeswitches.M8 := FALSE;
   TANK_No0010.PCONF.Modeswitches.M9 := FALSE;
   TANK_No0010.PCONF.Modeswitches.M10 := FALSE;
   TANK_No0010.PCONF.Modeswitches.M11 := FALSE;
   TANK_No0010.PCONF.Modeswitches.M12 := FALSE;
   TANK_No0010.PCONF.Modeswitches.M13 := FALSE;
   TANK_No0010.PCONF.Modeswitches.M14 := FALSE;
   TANK_No0010.PCONF.Modeswitches.M15 := FALSE;
END_DATA_BLOCK

